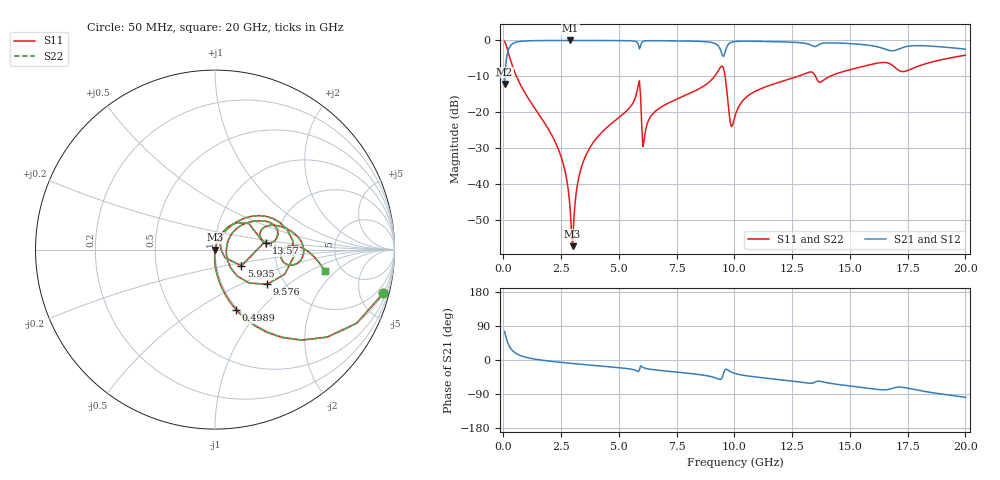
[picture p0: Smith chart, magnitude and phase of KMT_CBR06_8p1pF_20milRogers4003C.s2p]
! Data measured by Modelithics Inc. support@modelithics.com 813-866-6335
! KEMET CBR0603 8.1pF, Pad Width= 0.851mm, Pad Length= 0.64mm, Pad Gap= 0.62mm, 20mil Rogers 4003C substrate Data, January 2022
# hz S ma R 50
! 2 Port Network Data from SP1.SP block
! freq  magS11  angS11  magS21  angS21  magS12  angS12  magS22  angS22
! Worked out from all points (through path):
!   401 points, 50 MHz to 20 GHz, reference 50 ohm
!   highest |S21| = -0.01 dB at 2.893 GHz (marker M1); lowest = -12.1 dB at 50 MHz (marker M2)
!   group delay of S21, straight-line fit = 14.6 ps
!   lowest |S11| = -57.2 dB at 2.993 GHz (marker M3), VSWR 1.00, Z = 50.1 + j0.0273 ohm
!   |S11| at or under -10 dB: 564.6 MHz to 9.141 GHz (8.576 GHz wide, 177 % of centre); 9.594 GHz to 12.74 GHz (3.148 GHz wide, 28.2 % of centre); 13.51 GHz to 14.13 GHz (625.2 MHz wide, 4.52 % of centre)
!   |S22| runs from -57.2 to -0.3 dB; largest |S21 - S12| = 0
!   S11 on the Smith chart (normalised r, x): 50 MHz: 0.98, -7.72; 498.9 MHz: 0.98, -0.75; 5.935 GHz: 1.32, -0.25; 9.576 GHz: 1.62, -0.71; 13.57 GHz: 1.80, +0.15; 20 GHz: 3.69, -1.45
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5e7  0.9685 -14.5  0.2484 75.4  0.2484 75.4  0.9685 -14.5
2.495e8  0.6127 -52.9  0.7894 37.0  0.7894 37.0  0.6127 -52.9
4.98875e8  0.3552 -70.6  0.9339 19.3  0.9339 19.3  0.3552 -70.6
2.394125e9  0.0297 -93.5  0.9983 -5.7  0.9983 -5.7  0.0297 -93.5
2.693375e9  0.01384 -92.5  0.9986 -7.6  0.9986 -7.6  0.01384 -92.5
2.892875e9  0.004315 -81.7  0.9986 -8.7  0.9986 -8.7  0.004315 -81.7
2.992625e9  0.001377 11.4  0.9986 -9.3  0.9986 -9.3  0.001377 11.4
3.391625e9  0.01791 74.1  0.9983 -11.5  0.9983 -11.5  0.01791 74.1
5.785625e9  0.1962 49.9  0.9431 -29.0  0.9431 -29.0  0.1962 49.9
5.93525e9  0.1729 -31.7  0.8325 -15.6  0.8325 -15.6  0.1729 -31.7
6.084875e9  0.03948 40.7  0.9803 -20.8  0.9803 -20.8  0.03948 40.7
6.73325e9  0.1132 61.1  0.9901 -27.3  0.9901 -27.3  0.1132 61.1
9.177125e9  0.3277 34.9  0.9001 -47.1  0.9001 -47.1  0.3277 34.9
9.576125e9  0.3479 -33.6  0.6532 -27.2  0.6532 -27.2  0.3479 -33.6
9.8255e9  0.07029 -24.6  0.9297 -30.6  0.9297 -30.6  0.07029 -24.6
1.0025e10  0.08825 33.8  0.965 -35.5  0.965 -35.5  0.08825 33.8
1.0823e10  0.19 43.3  0.9727 -44.1  0.9727 -44.1  0.19 43.3
1.336662e10  0.3616 14.0  0.8437 -61.2  0.8437 -61.2  0.3616 14.0
1.356612e10  0.289 7.4  0.8374 -56.3  0.8374 -56.3  0.289 7.4
1.516212e10  0.4038 17.6  0.8962 -69.8  0.8962 -69.8  0.4038 17.6
1.670825e10  0.4773 -7.8  0.7253 -77.1  0.7253 -77.1  0.4773 -7.8
2e10  0.6228 -11.1  0.7547 -98.6  0.7547 -98.6  0.6228 -11.1
